FUNCTION_BLOCK "IMAC_MOTOR3_CALL"
TITLE =Function calls for MOTOR3 objects
//Parameter Description for Function MOTOR3 (FB82):
//-------------------------------------------------
//OBJ:     Ascending Object number for MOTOR3 (1...x)
//
//RMOT:    'REMOTE'     Feedback
//                      0 = Local
//                      1 = Remote)
//
//FWD:     'FORWARD'    Feedback 'Forward'
//                      0 = Not running in 'Forward Direction'
//                      1 = Running     in 'Forward Direction'
//
//BACK:    'REVERSE'    Feedback 'Reverse'
//                      0 = Not running in 'Reverse Direction'
//                      1 = Running     in 'Reverse Direction'
//
//SLOW:     'SLOW'      Feedback 'Low Speed'
//                      0 = Not running in 'Low Speed'
//                      1 = Running     in 'Low Speed'
//
//FAST:     'FAST'      Feedback 'Reverse'
//                      0 = Not running in 'High Speed'
//                      1 = Running     in 'High Speed'
//
//FAUL     'EXT. FAULT' Feedback. Function dep. on Mode Switch 'M10_ExtFaultNC':
//                      If 'M10_ExtFaultNC' = 0 :       0 = OK,    1 = Fault
//                      If 'M10_ExtFaultNC' = 1 :       0 = Fault, 1 = OK
//
//ACOM:    'AUTO' Mode  Command Interface (only active, if 'REMOTE'+'AUTO')
//                      Bit  0       : BlackoutStart Command
//                      Bit  7       : FetchData Command (from Standby Unit)
//                      Bit  8       : Start Command 'Forward+Slow'
//                      Bit  9       : Stop Command
//                      Bit 10       : Failure input from Automatic Function
//                      Bit 11       : Lock Start/Stop Commands
//                      Bit 12       : Emergency Off
//                      Bit 13       : Start Command 'Forward+Fast'
//                      Bit 14       : Start Command 'Reverse+Slow'
//                      Bit 15       : Start Command 'Reverse+Fast'
//
//BLKO:    'BLACKOUT'   Feedback
//                      0 = No Blackout
//                      1 = Blackout
//
//PCONF:   (leave empty, refers to local instance data in Instance DB)
//
//MFWD:    'START FWD'  Output to Motor 'Start Forward'
//                      0 = No Command
//                      1 = Start Command 'Forward'
//
//MBAC:    'START BACK' Output to Motor 'Start Reverse'
//                      0 = No Command
//                      1 = Start Command 'Reverse'
//
//MSLO:    'START SLOW' Output to Motor 'Start Slow'
//                      0 = No Command
//                      1 = Start Command 'Slow'
//
//MFAS:    'START FAST' Output to Motor 'Start Fast'
//                      0 = No Command
//                      1 = Start Command 'Fast'
//
//MSTO:    'STOP'       Output to Motor 'Stop'
//                      0 = No Command
//                      1 = Stop Command
//
//STAT:   'AUTO' Mode  Status Interface
//                      Bit  0       : Running 'Forward & Fast'
//                      Bit  1       : Running 'Reverse & Slow'
//                      Bit  2       : Running 'Reverse & Fast'
//                      Bit  8       : Running 'Forward & Slow'
//                      Bit  9       : Local
//                      Bit 10       : Manual
//                      Bit 11       : Auto
//                      Bit 12       : Failure
//                      Bit 13       : BlackOut
//                      Bit 14       : Starting
//                      Bit 15       : Restarting
//
//OSSTAT:  OS Status Word
//                      Value = 0    : Undefined
//                      Value = 1    : Running1 'Forward & Slow'
//                      Value = 2    : Running2 'Forward & Fast'
//                      Value = 3    : Running3 'Reverse & Slow'
//                      Value = 4    : Running4 'Reverse & Fast'
//                      Value = 5    : (not used)
//                      Value = 6    : Starting1 'Forward & Slow'
//                      Value = 7    : Starting2 'Forward & Fast'
//                      Value = 8    : Starting3 'Reverse & Slow'
//                      Value = 9    : Starting4 'Reverse & Fast'
//                      Value = 10   : Stopped
//                      Value = 11   : Blackout
//                      Value + 256  : Local Mode  (Offset Value)
//                      Value + 512  : Manual Mode (Offset Value)
//                      Value + 1024 : Auto Mode   (Offset Value)
//
//OSALARM: OS Alarm Word
//                      Value = 0    : Undefined
//                      Value = 1    : Normal
//                      Value = 2    : External Fault Alarm
//                      Value = 3    : Auto Failure Alarm
//                      Value = 4    : Action Alarm
//                      Value = 5    : Non-Feedback Alarm
//                      Value = 6    : Lock
//                      Value = 7    : Emergency Off
//                      Value = 8    : Blackout
//
//OSCOM:   OS Command Interface
//                      Bit  0       : Start1 'Forward & Slow' Command
//                      Bit  1       : Start2 'Forward & Fast' Command
//                      Bit  2       : Start2 'Reverse & Slow' Command
//                      Bit  3       : Start4 'Reverse & Fast' Command
//                      Bit  4       : Stop   Command
//                      Bit  7       : Reset  Command
//                      Bit  9       : Manual Command
//                      Bit 10       : Auto   Command
AUTHOR : Edelmann
FAMILY : IMAC
VERSION : 0.1


VAR
  MotorNo_001 : "IMAC_MOTOR3";
  MotorNo_002 : "IMAC_MOTOR3";
  MotorNo_003 : "IMAC_MOTOR3";
  MotorNo_004 : "IMAC_MOTOR3";
  MotorNo_005 : "IMAC_MOTOR3";
  MotorNo_006 : "IMAC_MOTOR3";
  MotorNo_007 : "IMAC_MOTOR3";
  MotorNo_008 : "IMAC_MOTOR3";
  MotorNo_009 : "IMAC_MOTOR3";
  MotorNo_010 : "IMAC_MOTOR3";
  MotorNo_011 : "IMAC_MOTOR3";
  MotorNo_012 : "IMAC_MOTOR3";
  MotorNo_013 : "IMAC_MOTOR3";
  MotorNo_014 : "IMAC_MOTOR3";
  MotorNo_015 : "IMAC_MOTOR3";
  MotorNo_016 : "IMAC_MOTOR3";
  MotorNo_017 : "IMAC_MOTOR3";
  MotorNo_018 : "IMAC_MOTOR3";
  MotorNo_019 : "IMAC_MOTOR3";
  MotorNo_020 : "IMAC_MOTOR3";
  MotorNo_021 : "IMAC_MOTOR3";
  MotorNo_022 : "IMAC_MOTOR3";
  MotorNo_023 : "IMAC_MOTOR3";
  MotorNo_024 : "IMAC_MOTOR3";
  MotorNo_025 : "IMAC_MOTOR3";
END_VAR
BEGIN
NETWORK
TITLE =MOTOR3 Number 001

      CALL #MotorNo_001 (
           OBJ                      := 1,
           RMOT                     := E      6.7,
           FWD                      := E      7.0,
           BACK                     := E      7.1,
           SLOW                     := E      7.2,
           FAST                     := E      7.3,
           FAUL                     := E      7.4,
           ACOM                     := "IMAC_MOTOR3_I/O".MOTOR3_001_ACOM,
           BLKO                     := E      7.5,
           MFWD                     := A      3.1,
           MBAC                     := A      3.2,
           MSLO                     := A      3.3,
           MFAS                     := A      3.4,
           MSTO                     := A      3.5,
           STAT                     := "IMAC_MOTOR3_I/O".MOTOR3_001_STAT,
           OSSTAT                   := "IMAC_MOTOR3_I/O".MOTOR3_001_OSSTAT,
           OSALARM                  := "IMAC_MOTOR3_I/O".MOTOR3_001_OSALARM,
           OSCOM                    := "IMAC_MOTOR3_I/O".MOTOR3_001_OSCOM);

NETWORK
TITLE =MOTOR3 Number 002

//*********** END of Function Processing ! *******************************************************************
      BEA   ; // Move this Instruction down to the next Network to add one object !
//************************************************************************************************************

      CALL #MotorNo_002 (
           OBJ                      := 2,
           ACOM                     := "IMAC_MOTOR3_I/O".MOTOR3_002_ACOM,
           STAT                     := "IMAC_MOTOR3_I/O".MOTOR3_002_STAT,
           OSSTAT                   := "IMAC_MOTOR3_I/O".MOTOR3_002_OSSTAT,
           OSALARM                  := "IMAC_MOTOR3_I/O".MOTOR3_002_OSALARM,
           OSCOM                    := "IMAC_MOTOR3_I/O".MOTOR3_002_OSCOM);

NETWORK
TITLE =MOTOR3 Number 003

      CALL #MotorNo_003 (
           OBJ                      := 3,
           ACOM                     := "IMAC_MOTOR3_I/O".MOTOR3_003_ACOM,
           STAT                     := "IMAC_MOTOR3_I/O".MOTOR3_003_STAT,
           OSSTAT                   := "IMAC_MOTOR3_I/O".MOTOR3_003_OSSTAT,
           OSALARM                  := "IMAC_MOTOR3_I/O".MOTOR3_003_OSALARM,
           OSCOM                    := "IMAC_MOTOR3_I/O".MOTOR3_003_OSCOM);

NETWORK
TITLE =MOTOR3 Number 004

      CALL #MotorNo_004 (
           OBJ                      := 4,
           ACOM                     := "IMAC_MOTOR3_I/O".MOTOR3_004_ACOM,
           STAT                     := "IMAC_MOTOR3_I/O".MOTOR3_004_STAT,
           OSSTAT                   := "IMAC_MOTOR3_I/O".MOTOR3_004_OSSTAT,
           OSALARM                  := "IMAC_MOTOR3_I/O".MOTOR3_004_OSALARM,
           OSCOM                    := "IMAC_MOTOR3_I/O".MOTOR3_004_OSCOM);

NETWORK
TITLE =MOTOR3 Number 005

      CALL #MotorNo_005 (
           OBJ                      := 5,
           ACOM                     := "IMAC_MOTOR3_I/O".MOTOR3_005_ACOM,
           STAT                     := "IMAC_MOTOR3_I/O".MOTOR3_005_STAT,
           OSSTAT                   := "IMAC_MOTOR3_I/O".MOTOR3_005_OSSTAT,
           OSALARM                  := "IMAC_MOTOR3_I/O".MOTOR3_005_OSALARM,
           OSCOM                    := "IMAC_MOTOR3_I/O".MOTOR3_005_OSCOM);

NETWORK
TITLE =MOTOR3 Number 006

      CALL #MotorNo_006 (
           OBJ                      := 6,
           ACOM                     := "IMAC_MOTOR3_I/O".MOTOR3_006_ACOM,
           STAT                     := "IMAC_MOTOR3_I/O".MOTOR3_006_STAT,
           OSSTAT                   := "IMAC_MOTOR3_I/O".MOTOR3_006_OSSTAT,
           OSALARM                  := "IMAC_MOTOR3_I/O".MOTOR3_006_OSALARM,
           OSCOM                    := "IMAC_MOTOR3_I/O".MOTOR3_006_OSCOM);

NETWORK
TITLE =MOTOR3 Number 007

      CALL #MotorNo_007 (
           OBJ                      := 7,
           ACOM                     := "IMAC_MOTOR3_I/O".MOTOR3_007_ACOM,
           STAT                     := "IMAC_MOTOR3_I/O".MOTOR3_007_STAT,
           OSSTAT                   := "IMAC_MOTOR3_I/O".MOTOR3_007_OSSTAT,
           OSALARM                  := "IMAC_MOTOR3_I/O".MOTOR3_007_OSALARM,
           OSCOM                    := "IMAC_MOTOR3_I/O".MOTOR3_007_OSCOM);

NETWORK
TITLE =MOTOR3 Number 008

      CALL #MotorNo_008 (
           OBJ                      := 8,
           ACOM                     := "IMAC_MOTOR3_I/O".MOTOR3_008_ACOM,
           STAT                     := "IMAC_MOTOR3_I/O".MOTOR3_008_STAT,
           OSSTAT                   := "IMAC_MOTOR3_I/O".MOTOR3_008_OSSTAT,
           OSALARM                  := "IMAC_MOTOR3_I/O".MOTOR3_008_OSALARM,
           OSCOM                    := "IMAC_MOTOR3_I/O".MOTOR3_008_OSCOM);

NETWORK
TITLE =MOTOR3 Number 009

      CALL #MotorNo_009 (
           OBJ                      := 9,
           ACOM                     := "IMAC_MOTOR3_I/O".MOTOR3_009_ACOM,
           STAT                     := "IMAC_MOTOR3_I/O".MOTOR3_009_STAT,
           OSSTAT                   := "IMAC_MOTOR3_I/O".MOTOR3_009_OSSTAT,
           OSALARM                  := "IMAC_MOTOR3_I/O".MOTOR3_009_OSALARM,
           OSCOM                    := "IMAC_MOTOR3_I/O".MOTOR3_009_OSCOM);

NETWORK
TITLE =MOTOR3 Number 010

      CALL #MotorNo_010 (
           OBJ                      := 10,
           ACOM                     := "IMAC_MOTOR3_I/O".MOTOR3_010_ACOM,
           STAT                     := "IMAC_MOTOR3_I/O".MOTOR3_010_STAT,
           OSSTAT                   := "IMAC_MOTOR3_I/O".MOTOR3_010_OSSTAT,
           OSALARM                  := "IMAC_MOTOR3_I/O".MOTOR3_010_OSALARM,
           OSCOM                    := "IMAC_MOTOR3_I/O".MOTOR3_010_OSCOM);

NETWORK
TITLE =MOTOR3 Number 011

      CALL #MotorNo_011 (
           OBJ                      := 11,
           ACOM                     := "IMAC_MOTOR3_I/O".MOTOR3_011_ACOM,
           STAT                     := "IMAC_MOTOR3_I/O".MOTOR3_011_STAT,
           OSSTAT                   := "IMAC_MOTOR3_I/O".MOTOR3_011_OSSTAT,
           OSALARM                  := "IMAC_MOTOR3_I/O".MOTOR3_011_OSALARM,
           OSCOM                    := "IMAC_MOTOR3_I/O".MOTOR3_011_OSCOM);

NETWORK
TITLE =MOTOR3 Number 012

      CALL #MotorNo_012 (
           OBJ                      := 12,
           ACOM                     := "IMAC_MOTOR3_I/O".MOTOR3_012_ACOM,
           STAT                     := "IMAC_MOTOR3_I/O".MOTOR3_012_STAT,
           OSSTAT                   := "IMAC_MOTOR3_I/O".MOTOR3_012_OSSTAT,
           OSALARM                  := "IMAC_MOTOR3_I/O".MOTOR3_012_OSALARM,
           OSCOM                    := "IMAC_MOTOR3_I/O".MOTOR3_012_OSCOM);

NETWORK
TITLE =MOTOR3 Number 013

      CALL #MotorNo_013 (
           OBJ                      := 13,
           ACOM                     := "IMAC_MOTOR3_I/O".MOTOR3_013_ACOM,
           STAT                     := "IMAC_MOTOR3_I/O".MOTOR3_013_STAT,
           OSSTAT                   := "IMAC_MOTOR3_I/O".MOTOR3_013_OSSTAT,
           OSALARM                  := "IMAC_MOTOR3_I/O".MOTOR3_013_OSALARM,
           OSCOM                    := "IMAC_MOTOR3_I/O".MOTOR3_013_OSCOM);

NETWORK
TITLE =MOTOR3 Number 014

      CALL #MotorNo_014 (
           OBJ                      := 14,
           ACOM                     := "IMAC_MOTOR3_I/O".MOTOR3_014_ACOM,
           STAT                     := "IMAC_MOTOR3_I/O".MOTOR3_014_STAT,
           OSSTAT                   := "IMAC_MOTOR3_I/O".MOTOR3_014_OSSTAT,
           OSALARM                  := "IMAC_MOTOR3_I/O".MOTOR3_014_OSALARM,
           OSCOM                    := "IMAC_MOTOR3_I/O".MOTOR3_014_OSCOM);

NETWORK
TITLE =MOTOR3 Number 015

      CALL #MotorNo_015 (
           OBJ                      := 15,
           ACOM                     := "IMAC_MOTOR3_I/O".MOTOR3_015_ACOM,
           STAT                     := "IMAC_MOTOR3_I/O".MOTOR3_015_STAT,
           OSSTAT                   := "IMAC_MOTOR3_I/O".MOTOR3_015_OSSTAT,
           OSALARM                  := "IMAC_MOTOR3_I/O".MOTOR3_015_OSALARM,
           OSCOM                    := "IMAC_MOTOR3_I/O".MOTOR3_015_OSCOM);

NETWORK
TITLE =MOTOR3 Number 016

      CALL #MotorNo_016 (
           OBJ                      := 16,
           ACOM                     := "IMAC_MOTOR3_I/O".MOTOR3_016_ACOM,
           STAT                     := "IMAC_MOTOR3_I/O".MOTOR3_016_STAT,
           OSSTAT                   := "IMAC_MOTOR3_I/O".MOTOR3_016_OSSTAT,
           OSALARM                  := "IMAC_MOTOR3_I/O".MOTOR3_016_OSALARM,
           OSCOM                    := "IMAC_MOTOR3_I/O".MOTOR3_016_OSCOM);

NETWORK
TITLE =MOTOR3 Number 017

      CALL #MotorNo_017 (
           OBJ                      := 17,
           ACOM                     := "IMAC_MOTOR3_I/O".MOTOR3_017_ACOM,
           STAT                     := "IMAC_MOTOR3_I/O".MOTOR3_017_STAT,
           OSSTAT                   := "IMAC_MOTOR3_I/O".MOTOR3_017_OSSTAT,
           OSALARM                  := "IMAC_MOTOR3_I/O".MOTOR3_017_OSALARM,
           OSCOM                    := "IMAC_MOTOR3_I/O".MOTOR3_017_OSCOM);

NETWORK
TITLE =MOTOR3 Number 018

      CALL #MotorNo_018 (
           OBJ                      := 18,
           ACOM                     := "IMAC_MOTOR3_I/O".MOTOR3_018_ACOM,
           STAT                     := "IMAC_MOTOR3_I/O".MOTOR3_018_STAT,
           OSSTAT                   := "IMAC_MOTOR3_I/O".MOTOR3_018_OSSTAT,
           OSALARM                  := "IMAC_MOTOR3_I/O".MOTOR3_018_OSALARM,
           OSCOM                    := "IMAC_MOTOR3_I/O".MOTOR3_018_OSCOM);

NETWORK
TITLE =MOTOR3 Number 019

      CALL #MotorNo_019 (
           OBJ                      := 19,
           ACOM                     := "IMAC_MOTOR3_I/O".MOTOR3_019_ACOM,
           STAT                     := "IMAC_MOTOR3_I/O".MOTOR3_019_STAT,
           OSSTAT                   := "IMAC_MOTOR3_I/O".MOTOR3_019_OSSTAT,
           OSALARM                  := "IMAC_MOTOR3_I/O".MOTOR3_019_OSALARM,
           OSCOM                    := "IMAC_MOTOR3_I/O".MOTOR3_019_OSCOM);

NETWORK
TITLE =MOTOR3 Number 020

      CALL #MotorNo_020 (
           OBJ                      := 20,
           ACOM                     := "IMAC_MOTOR3_I/O".MOTOR3_020_ACOM,
           STAT                     := "IMAC_MOTOR3_I/O".MOTOR3_020_STAT,
           OSSTAT                   := "IMAC_MOTOR3_I/O".MOTOR3_020_OSSTAT,
           OSALARM                  := "IMAC_MOTOR3_I/O".MOTOR3_020_OSALARM,
           OSCOM                    := "IMAC_MOTOR3_I/O".MOTOR3_020_OSCOM);

NETWORK
TITLE =MOTOR3 Number 021

      CALL #MotorNo_021 (
           OBJ                      := 21,
           ACOM                     := "IMAC_MOTOR3_I/O".MOTOR3_021_ACOM,
           STAT                     := "IMAC_MOTOR3_I/O".MOTOR3_021_STAT,
           OSSTAT                   := "IMAC_MOTOR3_I/O".MOTOR3_021_OSSTAT,
           OSALARM                  := "IMAC_MOTOR3_I/O".MOTOR3_021_OSALARM,
           OSCOM                    := "IMAC_MOTOR3_I/O".MOTOR3_021_OSCOM);

NETWORK
TITLE =MOTOR3 Number 022

      CALL #MotorNo_022 (
           OBJ                      := 22,
           ACOM                     := "IMAC_MOTOR3_I/O".MOTOR3_022_ACOM,
           STAT                     := "IMAC_MOTOR3_I/O".MOTOR3_022_STAT,
           OSSTAT                   := "IMAC_MOTOR3_I/O".MOTOR3_022_OSSTAT,
           OSALARM                  := "IMAC_MOTOR3_I/O".MOTOR3_022_OSALARM,
           OSCOM                    := "IMAC_MOTOR3_I/O".MOTOR3_022_OSCOM);

NETWORK
TITLE =MOTOR3 Number 023

      CALL #MotorNo_023 (
           OBJ                      := 23,
           ACOM                     := "IMAC_MOTOR3_I/O".MOTOR3_023_ACOM,
           STAT                     := "IMAC_MOTOR3_I/O".MOTOR3_023_STAT,
           OSSTAT                   := "IMAC_MOTOR3_I/O".MOTOR3_023_OSSTAT,
           OSALARM                  := "IMAC_MOTOR3_I/O".MOTOR3_023_OSALARM,
           OSCOM                    := "IMAC_MOTOR3_I/O".MOTOR3_023_OSCOM);

NETWORK
TITLE =MOTOR3 Number 024

      CALL #MotorNo_024 (
           OBJ                      := 24,
           ACOM                     := "IMAC_MOTOR3_I/O".MOTOR3_024_ACOM,
           STAT                     := "IMAC_MOTOR3_I/O".MOTOR3_024_STAT,
           OSSTAT                   := "IMAC_MOTOR3_I/O".MOTOR3_024_OSSTAT,
           OSALARM                  := "IMAC_MOTOR3_I/O".MOTOR3_024_OSALARM,
           OSCOM                    := "IMAC_MOTOR3_I/O".MOTOR3_024_OSCOM);

NETWORK
TITLE =MOTOR3 Number 025

      CALL #MotorNo_025 (
           OBJ                      := 25,
           ACOM                     := "IMAC_MOTOR3_I/O".MOTOR3_025_ACOM,
           STAT                     := "IMAC_MOTOR3_I/O".MOTOR3_025_STAT,
           OSSTAT                   := "IMAC_MOTOR3_I/O".MOTOR3_025_OSSTAT,
           OSALARM                  := "IMAC_MOTOR3_I/O".MOTOR3_025_OSALARM,
           OSCOM                    := "IMAC_MOTOR3_I/O".MOTOR3_025_OSCOM);

END_FUNCTION_BLOCK

